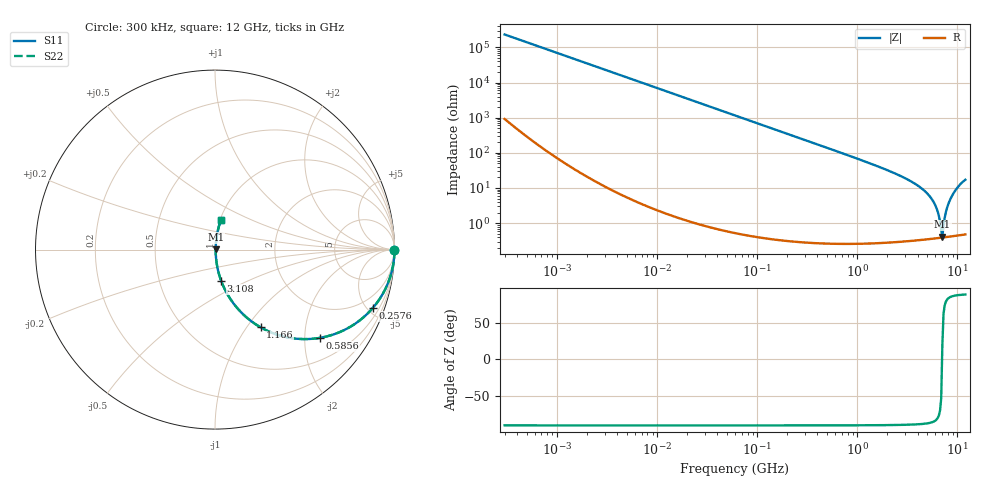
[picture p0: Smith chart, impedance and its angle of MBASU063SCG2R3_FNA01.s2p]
! MBASU063SCG2R3_FNA01  S-PARAMETER MODEL  ( General Type )
! Model Generated by TAIYO YUDEN Corporation (http://www.ty-top.com)
! Version 1.0
! TAIYO YUDEN Control No. 130801
! Copyright(c) 2013 TAIYO YUDEN CO.,LTD. All Rights Reserved.
! Product Description (link to TY-COMPAS)
! https://ds.yuden.co.jp/TYCOMPAS/or/detail?pn=MBASU063SCG2R3CFNA01&u=M
! Products Name : Multilayer Ceramic Capacitors
! Characteristics :
!  Capacitance : 2.3 pF , Rated Voltage : 50V , TCC : CG / C0G
!  Case Size : 0.6 x 0.3 / 0.024 x 0.012 [mm/inch] , Thickness : 0.3 / 0.012 [mm/inch]
!  (Conditions: Temperature = 25 degC , DC Bias Current/Voltage = 0A / 0V)
! External Node Assignments :
!  1  o---| |---o  2
! GND o---------o GND
! Frequency Range : 0.3MHz  -  12000MHz  [ 401 STEP ]
# MHz S RI R 50
! Freq[MHz].  S11 Real  S11 Imag  S21 Real  S21 Imag  S12 Real  S12 Imag  S22 Real  S22 Imag
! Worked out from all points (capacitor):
!   401 points, 300 kHz to 12 GHz, reference 50 ohm
!   read as one part in series: C = 2.28 pF near 316.3 kHz
!   lowest |Z| = 413 mohm at 7.064 GHz (marker M1)
!   series resonance near 7.026 GHz, so ESL is about 220 pH
!   S11 on the Smith chart (normalised r, x): 300 kHz: open; 257.6 MHz: 1.01, -5.40; 585.6 MHz: 1.01, -2.36; 1.166 GHz: 1.01, -1.16; 3.108 GHz: 1.01, -0.36; 12 GHz: 1.01, +0.34
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0.3  1 -0.00043  1.89e-06 0.00043  1.89e-06 0.00043  1 -0.00043
1.769972  1 -0.00254  8.1e-06 0.00254  8.1e-06 0.00254  1 -0.00254
10.44266  0.9998 -0.015  0.000229 0.015  0.000229 0.015  0.9998 -0.015
60  0.9926 -0.0854  0.00739 0.0854  0.00739 0.0854  0.9926 -0.0854
257.5933  0.8793 -0.3253  0.1207 0.3253  0.1207 0.3253  0.8793 -0.3253
353.9943  0.7938 -0.4039  0.2062 0.4039  0.2062 0.4039  0.7938 -0.4039
585.5907  0.5827 -0.492  0.4173 0.492  0.4173 0.492  0.5827 -0.492
1166.079  0.2536 -0.4328  0.7464 0.4328  0.7464 0.4328  0.2536 -0.4328
2088.533  0.087 -0.2773  0.913 0.2773  0.913 0.2773  0.087 -0.2773
3107.553  0.0344 -0.1741  0.9656 0.1741  0.9656 0.1741  0.0344 -0.1741
4385.161  0.0127 -0.096  0.9873 0.096  0.9873 0.096  0.0127 -0.096
5420.343  0.0063 -0.0522  0.9937 0.0522  0.9937 0.0522  0.0063 -0.0522
6026.253  0.00465 -0.0311  0.9953 0.0311  0.9953 0.0311  0.00465 -0.0311
6354.153  0.00417 -0.0206  0.9958 0.0206  0.9958 0.0206  0.00417 -0.0206
6699.894  0.00392 -0.0102  0.9961 0.0102  0.9961 0.0102  0.00392 -0.0102
6879.757  0.00387 -0.0051  0.9961 0.0051  0.9961 0.0051  0.00387 -0.0051
7064.448  0.00389 0.00134  0.9961 -0.00134  0.9961 -0.00134  0.00389 0.00134
7254.098  0.00398 0.00729  0.996 -0.00729  0.996 -0.00729  0.00398 0.00729
8064.993  0.00518 0.0332  0.9948 -0.0332  0.9948 -0.0332  0.00518 0.0332
8732.115  0.00734 0.0559  0.9927 -0.0559  0.9927 -0.0559  0.00734 0.0559
10236.47  0.0166 0.1093  0.9834 -0.1093  0.9834 -0.1093  0.0166 0.1093
12000  0.033 0.1653  0.967 -0.1653  0.967 -0.1653  0.033 0.1653
